|Texas Instruments Incorporated
|XWRL6888 Single-Chip 60GHz mmWave Sensor
[IBIS Ver]   5.0
[File name]   xwrl6888_fccsp329.ibs
[Date]   07/08/2026
[File Rev]   1.0
[Source]   Cadence SpeedXP Suite XtractIM 18.0.4.05011.160686   004
[Notes]   Revision History:
| Rev 1.0: 07/08/2026
| - Initial release of the model.
[Disclaimer]
| This model is designed as an aid for customers of Texas Instruments.
| TI and its licensors and suppliers make no warranties, either expressed
| or implied, with respect to this  model, including the warranties of
| merchantability or fitness for a particular purpose. The model is
| provided solely on an "as is" basis. The entire risk as to its quality
| and performance is with the customer.
| This model is subject to change without notice. Texas Instruments
| Incorporated is not responsible for updating this model.
[Copyright]
(C) Copyright 2021 Texas Instruments Incorporated.All rights reserved.
|  Component AWRL6888DBGAPDRQ1 329-pin FCBGA - APD0329 package
|  Part # AWRL6888DBGAPDRQ1
[Component]   AWRL6888DBGAPDRQ1
[Manufacturer]   Texas Instruments
[Package]   |329 FCCSP - APD0329 package
|  variable   typ   min   max
|   typ   min   max
R_pkg   0.17465   0.069398   0.39969
L_pkg   1.619e-9   6.542e-10   3.167e-9
C_pkg   5.691e-13   3.526e-13   1.287e-12
[Pin]   Signal_name   model_name   R_pin  L_pin  C_pin
A1   VSSA   GND   NA   NA   NA
A2   VSSA   GND   NA   NA   NA
A4   VSSA   GND   NA   NA   NA
A6   VSSA   GND   NA   NA   NA
A8   VSSA   GND   NA   NA   NA
A10   VSSA   GND   NA   NA   NA
A12   VSSA   GND   NA   NA   NA
A14   VSSA   GND   NA   NA   NA
A16   VSSA   GND   NA   NA   NA
A18   VSSA   GND   NA   NA   NA
A19   QSPI_qdin0   IO2   NA   NA   NA
A20   QSPI_qdin1   IO2   NA   NA   NA
A21   VSS   GND   NA   NA   NA
B1   VSSA   GND   NA   NA   NA
B2   VSSA   GND   NA   NA   NA
B3   TX1   NC   NA   NA   NA
B4   VSSA   GND   NA   NA   NA
B5   TX2   NC   NA   NA   NA
B6   VSSA   GND   NA   NA   NA
B7   TX3   NC   NA   NA   NA
B8   VSSA   GND   NA   NA   NA
B9   TX4   NC   NA   NA   NA
B10   VSSA   GND   NA   NA   NA
B11   TX5   NC   NA   NA   NA
B12   VSSA   GND   NA   NA   NA
B13   TX6   NC   NA   NA   NA
B14   VSSA   GND   NA   NA   NA
B15   TX7   NC   NA   NA   NA
B16   VSSA   GND   NA   NA   NA
B17   TX8   NC   NA   NA   NA
B18   VSSA   GND   NA   NA   NA
B19   VSS   GND   NA   NA   NA
B20   VSS   GND   NA   NA   NA
B21   QSPI_din   IO2   NA   NA   NA
C1   VSSA   GND   NA   NA   NA
C2   VSSA   GND   NA   NA   NA
C3   VSSA   GND   NA   NA   NA
C4   VSSA   GND   NA   NA   NA
C5   VSSA   GND   NA   NA   NA
C6   VSSA   GND   NA   NA   NA
C7   VSSA   GND   NA   NA   NA
C8   VSSA   GND   NA   NA   NA
C9   VSSA   GND   NA   NA   NA
C10   VSSA   GND   NA   NA   NA
C11   VSSA   GND   NA   NA   NA
C12   VSSA   GND   NA   NA   NA
C13   VSSA   GND   NA   NA   NA
C14   VSSA   GND   NA   NA   NA
C15   VSSA   GND   NA   NA   NA
C16   VSSA   GND   NA   NA   NA
C17   VSSA   GND   NA   NA   NA
C18   VSSA   GND   NA   NA   NA
C19   SPIA_miso   IO2   NA   NA   NA
C20   QSPI_dout   IO2   NA   NA   NA
C21   QSPI_cs_n   IO2   NA   NA   NA
D1   VSSA   GND   NA   NA   NA
D2   VSSA   GND   NA   NA   NA
D3   VSSA   GND   NA   NA   NA
D4   CLKM   NC   NA   NA   NA
D6   VSSA   GND   NA   NA   NA
D7   VSSA   GND   NA   NA   NA
D8   VSSA   GND   NA   NA   NA
D9   VSSA   GND   NA   NA   NA
D10   VSSA   GND   NA   NA   NA
D11   VSSA   GND   NA   NA   NA
D12   VSSA   GND   NA   NA   NA
D13   VSSA   GND   NA   NA   NA
D14   VSSA   GND   NA   NA   NA
D15   VSSA   GND   NA   NA   NA
D16   VSSA   GND   NA   NA   NA
D17   VSSA   GND   NA   NA   NA
D20   QSPI_clk   IO2   NA   NA   NA
E2   RX8   NC   NA   NA   NA
E3   VSSA   GND   NA   NA   NA
E19   SPIA_mosi   IO2   NA   NA   NA
E20   SPIA_cs0_n   IO2   NA   NA   NA
E21   PMIC_CLKOUT   IO2   NA   NA   NA
F1   VSSA   GND   NA   NA   NA
F2   VSSA   GND   NA   NA   NA
F3   VSSA   GND   NA   NA   NA
F4   CLKP   NC   NA   NA   NA
F6   VOUT_14SYNTH   NC   NA   NA   NA
F8   VDDA_10RF   POWER   NA   NA   NA
F9   VDDA_10RF   POWER   NA   NA   NA
F10   VDDA_10RF   POWER   NA   NA   NA
F11   VDDA_12RF   POWER   NA   NA   NA
F12   VDDA_12RF   POWER   NA   NA   NA
F13   VDDA_12RF   POWER   NA   NA   NA
F14   VSS   GND   NA   NA   NA
F15   VSS   GND   NA   NA   NA
F16   VSS   GND   NA   NA   NA
F19   SPIA_clk   IO2   NA   NA   NA
F20   VSS   GND   NA   NA   NA
F21   VIOIN_18   POWER   NA   NA   NA
G2   RX7   NC   NA   NA   NA
G3   VSSA   GND   NA   NA   NA
G8   VSSA   GND   NA   NA   NA
G9   VSSA   GND   NA   NA   NA
G10   VDD   POWER   NA   NA   NA
G11   VDD   POWER   NA   NA   NA
G12   VDD   POWER   NA   NA   NA
G13   VDD   POWER   NA   NA   NA
G14   VDD   POWER   NA   NA   NA
G15   VDD   POWER   NA   NA   NA
G16   VDD   POWER   NA   NA   NA
G20   VSS   GND   NA   NA   NA
G21   VIOIN   POWER   NA   NA   NA
H1   VSSA   GND   NA   NA   NA
H2   VSSA   GND   NA   NA   NA
H3   VSSA   GND   NA   NA   NA
H4   VSSA   GND   NA   NA   NA
H6   VIOIN_18CLK   POWER   NA   NA   NA
H8   OSC_CLK_OUT   NC   NA   NA   NA
H9   VSSA   GND   NA   NA   NA
H10   VDD   POWER   NA   NA   NA
H11   VDD   POWER   NA   NA   NA
H12   VDD   POWER   NA   NA   NA
H13   VDD   POWER   NA   NA   NA
H14   VDD   POWER   NA   NA   NA
H15   VDD   POWER   NA   NA   NA
H16   VDD   POWER   NA   NA   NA
H19   HOST_CLK_req   IO2   NA   NA   NA
H20   GPIO_2   IO2   NA   NA   NA
J2   RX6   NC   NA   NA   NA
J3   VSSA   GND   NA   NA   NA
J4   VSSA   GND   NA   NA   NA
J8   VSSA   GND   NA   NA   NA
J9   VSSA   GND   NA   NA   NA
J10   VDD   POWER   NA   NA   NA
J11   VDD   POWER   NA   NA   NA
J12   VDD   POWER   NA   NA   NA
J13   VDD   POWER   NA   NA   NA
J14   VDD   POWER   NA   NA   NA
J15   VDD   POWER   NA   NA   NA
J16   VDD   POWER   NA   NA   NA
J19   VSS   GND   NA   NA   NA
J20   LVDS_TXP0   ODF   NA   NA   NA
J21   LVDS_TXM0   ODF   NA   NA   NA
K1   VSSA   GND   NA   NA   NA
K2   VSSA   GND   NA   NA   NA
K3   VSSA   GND   NA   NA   NA
K4   VSSA   GND   NA   NA   NA
K6   VDDA_18VCO   POWER   NA   NA   NA
K8   VOUT_14APLL   NC   NA   NA   NA
K9   VSSA   GND   NA   NA   NA
K10   VDD   POWER   NA   NA   NA
K11   VDD   POWER   NA   NA   NA
K12   VDD   POWER   NA   NA   NA
K13   VDD   POWER   NA   NA   NA
K14   VDD   POWER   NA   NA   NA
K15   VDD   POWER   NA   NA   NA
K16   VDD   POWER   NA   NA   NA
K19   VSS   GND   NA   NA   NA
K20   LVDS_CLKP   ODF   NA   NA   NA
L2   RX5   NC   NA   NA   NA
L3   VSSA   GND   NA   NA   NA
L4   VSSA   GND   NA   NA   NA
L8   VSSA   GND   NA   NA   NA
L9   VSSA   GND   NA   NA   NA
L10   VDD   POWER   NA   NA   NA
L11   VDD   POWER   NA   NA   NA
L12   VDD   POWER   NA   NA   NA
L13   VDD   POWER   NA   NA   NA
L14   VDD   POWER   NA   NA   NA
L15   VDD   POWER   NA   NA   NA
L16   VDD   POWER   NA   NA   NA
L19   VSS   GND   NA   NA   NA
L20   VSS   GND   NA   NA   NA
L21   LVDS_CLKM   ODF   NA   NA   NA
M1   VSSA   GND   NA   NA   NA
M2   VSSA   GND   NA   NA   NA
M3   VSSA   GND   NA   NA   NA
M4   VSSA   GND   NA   NA   NA
M6   VIN_18PM   POWER   NA   NA   NA
M7   VDDA_10RF   POWER   NA   NA   NA
M8   VSSA   GND   NA   NA   NA
M9   VSS   GND   NA   NA   NA
M10   VSS   GND   NA   NA   NA
M11   VSS   GND   NA   NA   NA
M12   VSS   GND   NA   NA   NA
M13   VSS   GND   NA   NA   NA
M14   VSS   GND   NA   NA   NA
M15   VSS   GND   NA   NA   NA
M16   VSS   GND   NA   NA   NA
M19   VIOIN_18LVDS   POWER   NA   NA   NA
M20   VIOIN_18LVDS   POWER   NA   NA   NA
M21   LVDS_FRCLKM   ODF   NA   NA   NA
N2   RX4   NC   NA   NA   NA
N3   VSSA   GND   NA   NA   NA
N4   VSSA   GND   NA   NA   NA
N7   VSSA   GND   NA   NA   NA
N8   VSSA   GND   NA   NA   NA
N9   VSS   GND   NA   NA   NA
N10   VSS   GND   NA   NA   NA
N11   VSS   GND   NA   NA   NA
N12   VSS   GND   NA   NA   NA
N13   VSS   GND   NA   NA   NA
N14   VSS   GND   NA   NA   NA
N15   VSS   GND   NA   NA   NA
N16   VSS   GND   NA   NA   NA
N19   VSS   GND   NA   NA   NA
N20   LVDS_FRCLKP   ODF   NA   NA   NA
P1   VSSA   GND   NA   NA   NA
P2   VSSA   GND   NA   NA   NA
P3   VSSA   GND   NA   NA   NA
P4   VSSA   GND   NA   NA   NA
P6   VBGAP   NC   NA   NA   NA
P7   VSSA   GND   NA   NA   NA
P8   VSSA   GND   NA   NA   NA
P9   VSS   GND   NA   NA   NA
P10   VSS   GND   NA   NA   NA
P11   VSS   GND   NA   NA   NA
P12   VSS   GND   NA   NA   NA
P13   VSS   GND   NA   NA   NA
P14   VSS   GND   NA   NA   NA
P15   VSS   GND   NA   NA   NA
P16   VSS   GND   NA   NA   NA
P19   VSS   GND   NA   NA   NA
P20   LVDS_TXP1   ODF   NA   NA   NA
P21   LVDS_TXM1   ODF   NA   NA   NA
R2   RX3   NC   NA   NA   NA
R3   VSSA   GND   NA   NA   NA
R4   VSSA   GND   NA   NA   NA
R7   VSSA   GND   NA   NA   NA
R8   VSSA   GND   NA   NA   NA
R9   VSS   GND   NA   NA   NA
R10   VSS   GND   NA   NA   NA
R11   VSS   GND   NA   NA   NA
R12   VSS   GND   NA   NA   NA
R13   VSS   GND   NA   NA   NA
R14   VSS   GND   NA   NA   NA
R15   VSS   GND   NA   NA   NA
R16   VSS   GND   NA   NA   NA
R19   VSS   GND   NA   NA   NA
R20   I2C_sda   IO2   NA   NA   NA
T1   VSSA   GND   NA   NA   NA
T2   VSSA   GND   NA   NA   NA
T3   VSSA   GND   NA   NA   NA
T4   VSSA   GND   NA   NA   NA
T7   VSS   GND   NA   NA   NA
T8   VSS   GND   NA   NA   NA
T9   VSS   GND   NA   NA   NA
T10   VSS   GND   NA   NA   NA
T11   VSS   GND   NA   NA   NA
T12   VSS   GND   NA   NA   NA
T13   VSS   GND   NA   NA   NA
T14   VSS   GND   NA   NA   NA
T15   VSS   GND   NA   NA   NA
T16   VSS   GND   NA   NA   NA
T19   VSS   GND   NA   NA   NA
T20   lvds_valid   IO2   NA   NA   NA
T21   I2C_scl   IO2   NA   NA   NA
U2   RX2   NC   NA   NA   NA
U3   VSSA   GND   NA   NA   NA
U4   VSSA   GND   NA   NA   NA
U6   VSS   GND   NA   NA   NA
U7   VSS   GND   NA   NA   NA
U8   VSS   GND   NA   NA   NA
U9   VSS   GND   NA   NA   NA
U10   VSS   GND   NA   NA   NA
U11   VSS   GND   NA   NA   NA
U12   VSS   GND   NA   NA   NA
U13   VSS   GND   NA   NA   NA
U14   VSS   GND   NA   NA   NA
U15   VSS   GND   NA   NA   NA
U16   VSS   GND   NA   NA   NA
U19   VSS   GND   NA   NA   NA
U20   rs232_tx   IO2   NA   NA   NA
U21   sys_reset_out   IO2   NA   NA   NA
V1   VSSA   GND   NA   NA   NA
V2   VSSA   GND   NA   NA   NA
V3   VSSA   GND   NA   NA   NA
V6   VSS   GND   NA   NA   NA
V7   VSS   GND   NA   NA   NA
V8   VSS   GND   NA   NA   NA
V9   VSS   GND   NA   NA   NA
V12   VSS   GND   NA   NA   NA
V13   VSS   GND   NA   NA   NA
V14   VSS   GND   NA   NA   NA
V15   VSS   GND   NA   NA   NA
V16   VSS   GND   NA   NA   NA
V19   VSS   GND   NA   NA   NA
V20   rs232_rx   IO2   NA   NA   NA
W2   RX1   NC   NA   NA   NA
W3   VSSA   GND   NA   NA   NA
W6   VSS   GND   NA   NA   NA
W7   VSS   GND   NA   NA   NA
W8   VSS   GND   NA   NA   NA
W9   VSS   GND   NA   NA   NA
W19   VSS   GND   NA   NA   NA
W20   VSS   GND   NA   NA   NA
W21   VIOIN   POWER   NA   NA   NA
Y1   VSSA   GND   NA   NA   NA
Y2   VSSA   GND   NA   NA   NA
Y3   VSSA   GND   NA   NA   NA
Y4   VDDA_18BB   POWER   NA   NA   NA
Y5   GPADC4   NC   NA   NA   NA
Y6   VPP   POWER   NA   NA   NA
Y7   NRESET   NC   NA   NA   NA
Y8   UARTA_rx   IO1   NA   NA   NA
Y9   VDD   POWER   NA   NA   NA
Y10   VNWA   POWER   NA   NA   NA
Y11   VSS   GND   NA   NA   NA
Y12   VSS   GND   NA   NA   NA
Y13   VDD_SRAM   POWER   NA   NA   NA
Y14   TCK   IO1   NA   NA   NA
Y15   TDO   IO1   NA   NA   NA
Y16   TMS   IO1   NA   NA   NA
Y17   TDI   IO1   NA   NA   NA
Y18   LIN_tx   IO1   NA   NA   NA
Y19   GPIO_5   IO2   NA   NA   NA
Y20   VSS   GND   NA   NA   NA
Y21   VIOIN_18   POWER   NA   NA   NA
AA1   VSSA   GND   NA   NA   NA
AA2   GPADC1   NC   NA   NA   NA
AA3   GPADC2   NC   NA   NA   NA
AA4   VDDA_18BB   POWER   NA   NA   NA
AA6   GPADC3   NC   NA   NA   NA
AA7   UARTA_tx   IO1   NA   NA   NA
AA9   VDD   POWER   NA   NA   NA
AA10   VIOIN_18   POWER   NA   NA   NA
AA12   VIOIN   POWER   NA   NA   NA
AA13   VDD_SRAM   POWER   NA   NA   NA
AA14   CAN_FD_B_tx   IO1   NA   NA   NA
AA16   CAN_FD_B_rx   IO1   NA   NA   NA
AA17   LIN_rx   IO1   NA   NA   NA
AA19   UARTA_rts   IO2   NA   NA   NA
AA20   nERROR_OUT   IO2   NA   NA   NA
AA21   VSS   GND   NA   NA   NA
[Diff Pin]  inv_pin  vdiff  tdelay_typ  tdelay_min  tdelay_max
   P21   P20   0.1   NA   NA   NA
   M21   N20   0.1   NA   NA   NA
   L21   K20   0.1   NA   NA   NA
   J21   J20   0.1   NA   NA   NA
| Model IO1
[Model Selector] IO1
|SC1 IS A SLEW RATE CONTROL PIN
|5% SUPPLY VARIATION MODES WITH 1.8V NOM SUPPLY
IO1_V_PUPDOFF_5P_SC1_1P8  Cell operated at 1.8(nom)
|IO1_V_PUPDOFF_5P_SC1_1P8; BUFFER WITH WEAK PULUP/PULLDOWN OFF AT 5% SUPPLY
|VARIATION WITH SC1=1 MEANING SLOW MODE OF OPERATION
IO1_V_PD_ON_5P_!SC1_1P8  Cell operated at 1.8(nom)
|IO1_V_PD_ON_5P_!SC1_1P8; BUFFER WITH WEAK_PULLDOWN_ON AT 5% SUPPLY
|VARIATION WITH SC1=0 MEANING FAST MODE OF OPERATION
IO1_V_PD_ON_5P_SC1_1P8  Cell operated at 1.8(nom)
|IO1_V_PD_ON_5P_SC1_1P8; BUFFER WITH WEAK_PULLDOWN_ON AT 5% SUPPLY
|VARIATION WITH SC1=1 MEANING SLOW MODE OF OPERATION
IO1_V_PU_ON_5P_!SC1_1P8  Cell operated at 1.8(nom)
|IO1_V_PU_ON_5P_!SC1_1P8; BUFFER WITH WEAK_PULLUP_ON AT 5% SUPPLY
|VARIATION WITH SC1=0 MEANING FAST MODE OF OPERATION
IO1_V_PUPDOFF_5P_!SC1_1P8  Cell operated at 1.8(nom)
|IO1_V_PUPDOFF_5P_!SC1_1P8; BUFFER WITH WEAK PULUP/PULLDOWN OFF AT 5% SUPPLY
|VARIATION WITH SC1=0 MEANING FAST MODE OF OPERATION
IO1_V_PU_ON_5P_SC1_1P8  Cell operated at 1.8(nom)
|IO1_V_PU_ON_5P_SC1_1P8; BUFFER WITH WEAK_PULLUP_ON AT 5% SUPPLY
|VARIATION WITH SC1=1 MEANING SLOW MODE OF OPERATION
|5% SUPPLY VARIATION MODES WITH 3.3V NOM SUPPLY
IO1_V_PUPDOFF_5P_SC1_3P3  Cell operated at 3.3(nom)
|IO1_V_PUPDOFF_5P_SC1_3P3; BUFFER WITH WEAK PULUP/PULLDOWN OFF AT 5% SUPPLY
|VARIATION WITH SC1=1 MEANING SLOW MODE OF OPERATION
IO1_V_PD_ON_5P_!SC1_3P3  Cell operated at 3.3(nom)
|IO1_V_PD_ON_5P_!SC1_3P3; BUFFER WITH WEAK_PULLDOWN_ON AT 5% SUPPLY
|VARIATION WITH SC1=0 MEANING FAST MODE OF OPERATION
IO1_V_PD_ON_5P_SC1_3P3  Cell operated at 3.3(nom)
|IO1_V_PD_ON_5P_SC1_3P3; BUFFER WITH WEAK_PULLDOWN_ON AT 5% SUPPLY
|VARIATION WITH SC1=1 MEANING SLOW MODE OF OPERATION
IO1_V_PU_ON_5P_!SC1_3P3  Cell operated at 3.3(nom)
|IO1_V_PU_ON_5P_!SC1_3P3; BUFFER WITH WEAK_PULLUP_ON AT 5% SUPPLY
|VARIATION WITH SC1=0 MEANING FAST MODE OF OPERATION
IO1_V_PUPDOFF_5P_!SC1_3P3  Cell operated at 3.3(nom)
|IO1_V_PUPDOFF_5P_!SC1_3P3; BUFFER WITH WEAK PULUP/PULLDOWN OFF AT 5% SUPPLY
|VARIATION WITH SC1=0 MEANING FAST MODE OF OPERATION
IO1_V_PU_ON_5P_SC1_3P3  Cell operated at 3.3(nom)
|IO1_V_PU_ON_5P_SC1_3P3; BUFFER WITH WEAK_PULLUP_ON AT 5% SUPPLY
|VARIATION WITH SC1=1 MEANING SLOW MODE OF OPERATION
| 10% SUPPLY VARIATION MODES WITH 1.8V NOM SUPPLY
IO1_V_PUPDOFF_10P_SC1_1P8  Cell operated at 1.8(nom)
|IO1_V_PUPDOFF_10P_SC1_1P8; BUFFER WITH WEAK PULUP/PULLDOWN OFF AT 10% SUPPLY
|VARIATION WITH SC1=1 MEANING SLOW MODE OF OPERATION
IO1_V_PD_ON_10P_!SC1_1P8  Cell operated at 1.8(nom)
|IO1_V_PD_ON_10P_!SC1_1P8; BUFFER WITH WEAK_PULLDOWN_ON AT 10% SUPPLY
|VARIATION WITH SC1=0 MEANING FAST MODE OF OPERATION
IO1_V_PD_ON_10P_SC1_1P8  Cell operated at 1.8(nom)
|IO1_V_PD_ON_10P_SC1_1P8; BUFFER WITH WEAK_PULLDOWN_ON AT 10% SUPPLY
|VARIATION WITH SC1=1 MEANING SLOW MODE OF OPERATION
IO1_V_PU_ON_10P_!SC1_1P8  Cell operated at 1.8(nom)
|IO1_V_PU_ON_10P_!SC1_1P8; BUFFER WITH WEAK_PULLUP_ON AT 10% SUPPLY
|VARIATION WITH SC1=0 MEANING FAST MODE OF OPERATION
IO1_V_PUPDOFF_10P_!SC1_1P8  Cell operated at 1.8(nom)
|IO1_V_PUPDOFF_10P_!SC1_1P8; BUFFER WITH WEAK PULUP/PULLDOWN OFF AT 10% SUPPLY
|VARIATION WITH SC1=0 MEANING FAST MODE OF OPERATION
IO1_V_PU_ON_10P_SC1_1P8  Cell operated at 1.8(nom)
|IO1_V_PU_ON_10P_SC1_1P8; BUFFER WITH WEAK_PULLUP_ON AT 10% SUPPLY
|VARIATION WITH SC1=1 MEANING SLOW MODE OF OPERATION
| 10% SUPPLY VARIATION MODES WITH 3.3V NOM SUPPLY
IO1_V_PUPDOFF_10P_SC1_3P3  Cell operated at 3.3(nom)
|IO1_V_PUPDOFF_10P_SC1_3P3; BUFFER WITH WEAK PULUP/PULLDOWN OFF AT 10% SUPPLY
|VARIATION WITH SC1=1 MEANING SLOW MODE OF OPERATION
IO1_V_PD_ON_10P_!SC1_3P3  Cell operated at 3.3(nom)
|IO1_V_PD_ON_10P_!SC1_3P3; BUFFER WITH WEAK_PULLDOWN_ON 10% SUPPLY
|VARIATION WITH SC1=0 MEANING FAST MODE OF OPERATION
IO1_V_PD_ON_10P_SC1_3P3  Cell operated at 3.3(nom)
|IO1_V_PD_ON_10P_SC1_3P3; BUFFER WITH WEAK_PULLDOWN_ON AT 10% SUPPLY
|VARIATION WITH SC1=1 MEANING SLOW MODE OF OPERATION
IO1_V_PU_ON_10P_!SC1_3P3  Cell operated at 3.3(nom)
|IO1_V_PU_ON_10P_!SC1_3P3; BUFFER WITH WEAK_PULLUP_ON AT 10% SUPPLY
|VARIATION WITH SC1=0 MEANING FAST MODE OF OPERATION
IO1_V_PUPDOFF_10P_!SC1_3P3  Cell operated at 3.3(nom)
|IO1_V_PUPDOFF_10P_!SC1_3P3; BUFFER WITH WEAK PULUP/PULLDOWN OFF AT 10% SUPPLY
|VARIATION WITH SC1=0 MEANING FAST MODE OF OPERATION
IO1_V_PU_ON_10P_SC1_3P3  Cell operated at 3.3(nom)
|IO1_V_PU_ON_10P_SC1_3P3; BUFFER WITH WEAK_PULLUP_ON AT 10% SUPPLY
|VARIATION WITH SC1=1 MEANING SLOW MODE OF OPERATION
| Model IO2
[Model Selector] IO2
|SC1 IS A SLEW RATE CONTROL PIN
|5% SUPPLY VARIATION MODES WITH 1.8V NOM SUPPLY
IO2_H_PUPDOFF_5P_SC1_1P8  Cell operated at 1.8(nom)
|IO2_H_PUPDOFF_5P_SC1_1P8; BUFFER WITH WEAK PULUP/PULLDOWN OFF AT 5% SUPPLY
|VARIATION WITH SC1=1 MEANING SLOW MODE OF OPERATION
IO2_H_PD_ON_5P_!SC1_1P8  Cell operated at 1.8(nom)
|IO2_H_PD_ON_5P_!SC1_1P8; BUFFER WITH WEAK_PULLDOWN_ON AT 5% SUPPLY
|VARIATION WITH SC1=0 MEANING FAST MODE OF OPERATION
IO2_H_PD_ON_5P_SC1_1P8  Cell operated at 1.8(nom)
|IO2_H_PD_ON_5P_SC1_1P8; BUFFER WITH WEAK_PULLDOWN_ON AT 5% SUPPLY
|VARIATION WITH SC1=1 MEANING SLOW MODE OF OPERATION
IO2_H_PU_ON_5P_!SC1_1P8  Cell operated at 1.8(nom)
|IO2_H_PU_ON_5P_!SC1_1P8; BUFFER WITH WEAK_PULLUP_ON AT 5% SUPPLY
|VARIATION WITH SC1=0 MEANING FAST MODE OF OPERATION
IO2_H_PUPDOFF_5P_!SC1_1P8  Cell operated at 1.8(nom)
|IO2_H_PUPDOFF_5P_!SC1_1P8; BUFFER WITH WEAK PULUP/PULLDOWN OFF AT 5% SUPPLY
|VARIATION WITH SC1=0 MEANING FAST MODE OF OPERATION
IO2_H_PU_ON_5P_SC1_1P8  Cell operated at 1.8(nom)
|IO2_H_PU_ON_5P_SC1_1P8; BUFFER WITH WEAK_PULLUP_ON AT 5% SUPPLY
|VARIATION WITH SC1=1 MEANING SLOW MODE OF OPERATION
|5% SUPPLY VARIATION MODES WITH 3.3V NOM SUPPLY
IO2_H_PUPDOFF_5P_SC1_3P3  Cell operated at 3.3(nom)
|IO2_H_PUPDOFF_5P_SC1_3P3; BUFFER WITH WEAK PULUP/PULLDOWN OFF AT 5% SUPPLY
|VARIATION WITH SC1=1 MEANING SLOW MODE OF OPERATION
IO2_H_PD_ON_5P_!SC1_3P3  Cell operated at 3.3(nom)
|IO2_H_PD_ON_5P_!SC1_3P3; BUFFER WITH WEAK_PULLDOWN_ON AT 5% SUPPLY
|VARIATION WITH SC1=0 MEANING FAST MODE OF OPERATION
IO2_H_PD_ON_5P_SC1_3P3  Cell operated at 3.3(nom)
|IO2_H_PD_ON_5P_SC1_3P3; BUFFER WITH WEAK_PULLDOWN_ON AT 5% SUPPLY
|VARIATION WITH SC1=1 MEANING SLOW MODE OF OPERATION
IO2_H_PU_ON_5P_!SC1_3P3  Cell operated at 3.3(nom)
|IO2_H_PU_ON_5P_!SC1_3P3; BUFFER WITH WEAK_PULLUP_ON AT 5% SUPPLY
|VARIATION WITH SC1=0 MEANING FAST MODE OF OPERATION
IO2_H_PUPDOFF_5P_!SC1_3P3  Cell operated at 3.3(nom)
|IO2_H_PUPDOFF_5P_!SC1_3P3; BUFFER WITH WEAK PULUP/PULLDOWN OFF AT 5% SUPPLY
|VARIATION WITH SC1=0 MEANING FAST MODE OF OPERATION
IO2_H_PU_ON_5P_SC1_3P3  Cell operated at 3.3(nom)
|IO2_H_PU_ON_5P_SC1_3P3; BUFFER WITH WEAK_PULLUP_ON AT 5% SUPPLY
|VARIATION WITH SC1=1 MEANING SLOW MODE OF OPERATION
| 10% SUPPLY VARIATION MODES WITH 1.8V NOM SUPPLY
IO2_H_PUPDOFF_10P_SC1_1P8  Cell operated at 1.8(nom)
|IO2_H_PUPDOFF_10P_SC1_1P8; BUFFER WITH WEAK PULUP/PULLDOWN OFF AT 10% SUPPLY
|VARIATION WITH SC1=1 MEANING SLOW MODE OF OPERATION
IO2_H_PD_ON_10P_!SC1_1P8  Cell operated at 1.8(nom)
|IO2_H_PD_ON_10P_!SC1_1P8; BUFFER WITH WEAK_PULLDOWN_ON AT 10% SUPPLY
|VARIATION WITH SC1=0 MEANING FAST MODE OF OPERATION
IO2_H_PD_ON_10P_SC1_1P8  Cell operated at 1.8(nom)
|IO2_H_PD_ON_10P_SC1_1P8; BUFFER WITH WEAK_PULLDOWN_ON AT 10% SUPPLY
|VARIATION WITH SC1=1 MEANING SLOW MODE OF OPERATION
IO2_H_PU_ON_10P_!SC1_1P8  Cell operated at 1.8(nom)
|IO2_H_PU_ON_10P_!SC1_1P8; BUFFER WITH WEAK_PULLUP_ON AT 10% SUPPLY
|VARIATION WITH SC1=0 MEANING FAST MODE OF OPERATION
IO2_H_PUPDOFF_10P_!SC1_1P8  Cell operated at 1.8(nom)
|IO2_H_PUPDOFF_10P_!SC1_1P8; BUFFER WITH WEAK PULUP/PULLDOWN OFF AT 10% SUPPLY
|VARIATION WITH SC1=0 MEANING FAST MODE OF OPERATION
IO2_H_PU_ON_10P_SC1_1P8  Cell operated at 1.8(nom)
|IO2_H_PU_ON_10P_SC1_1P8; BUFFER WITH WEAK_PULLUP_ON AT 10% SUPPLY
|VARIATION WITH SC1=1 MEANING SLOW MODE OF OPERATION
| 10% SUPPLY VARIATION MODES WITH 3.3V NOM SUPPLY
IO2_H_PUPDOFF_10P_SC1_3P3  Cell operated at 3.3(nom)
|IO2_H_PUPDOFF_10P_SC1_3P3; BUFFER WITH WEAK PULUP/PULLDOWN OFF AT 10% SUPPLY
|VARIATION WITH SC1=1 MEANING SLOW MODE OF OPERATION
IO2_H_PD_ON_10P_!SC1_3P3  Cell operated at 3.3(nom)
|IO2_H_PD_ON_10P_!SC1_3P3; BUFFER WITH WEAK_PULLDOWN_ON 10% SUPPLY
|VARIATION WITH SC1=0 MEANING FAST MODE OF OPERATION
IO2_H_PD_ON_10P_SC1_3P3  Cell operated at 3.3(nom)
|IO2_H_PD_ON_10P_SC1_3P3; BUFFER WITH WEAK_PULLDOWN_ON AT 10% SUPPLY
|VARIATION WITH SC1=1 MEANING SLOW MODE OF OPERATION
IO2_H_PU_ON_10P_!SC1_3P3  Cell operated at 3.3(nom)
|IO2_H_PU_ON_10P_!SC1_3P3; BUFFER WITH WEAK_PULLUP_ON AT 10% SUPPLY
|VARIATION WITH SC1=0 MEANING FAST MODE OF OPERATION
IO2_H_PUPDOFF_10P_!SC1_3P3  Cell operated at 3.3(nom)
|IO2_H_PUPDOFF_10P_!SC1_3P3; BUFFER WITH WEAK PULUP/PULLDOWN OFF AT 10% SUPPLY
|VARIATION WITH SC1=0 MEANING FAST MODE OF OPERATION
IO2_H_PU_ON_10P_SC1_3P3  Cell operated at 3.3(nom)
|IO2_H_PU_ON_10P_SC1_3P3; BUFFER WITH WEAK_PULLUP_ON AT 10% SUPPLY
|VARIATION WITH SC1=1 MEANING SLOW MODE OF OPERATION
| Model ODF
[Model Selector] ODF
ODF_MODE_10P_1P8  Cell operated at 1.8(nom)
|ODF_MODE_10P_1P8; LVDS DRIVER MODE WITH 10PER VDDS
ODF_MODE_5P_1P8  Cell operated at 1.8(nom)
[Define Package Model]   AWRL6888DBGAPDRQ1
[Manufacturer]   TI
[OEM]   TI
[Description]   FCBGA
|[Number of Sections]   1
[Number of Pins]   64
[Pin Numbers]
|[Pin Name]  Net Number   Net Name   Net's All Pins
D4   | 1   CLKM   D4
F4   | 2   CLKP   F4
H8   | 3   OSC_CLK_OUT   H8
P6   | 4   VBGAP   P6
AA9   | 5   VDD   AA9
   |G10
   |G11
   |G12
   |G13
   |G14
   |G15
   |G16
   |H10
   |H11
   |H12
   |H13
   |H14
   |H15
   |H16
   |J10
   |J11
   |J12
   |J13
   |J14
   |J15
   |J16
   |K10
   |K11
   |K12
   |K13
   |K14
   |K15
   |K16
   |L10
   |L11
   |L12
   |L13
   |L14
   |L15
   |L16
   |Y9
F8   | 6   VDDA_10RF   F8
   |F9
   |F10
   |M7
F11   | 7   VDDA_12RF   F11
   |F12
   |F13
AA4   | 8   VDDA_18BB   AA4
   |Y4
K6   | 9   VDDA_18VCO   K6
AA13   | 10   VDD_SRAM   AA13
   |Y13
M6   | 11   VIN_18PM   M6
AA12   | 12   VIOIN   AA12
   |G21
   |W21
AA10   | 13   VIOIN_18   AA10
   |F21
   |Y21
H6   | 14   VIOIN_18CLK   H6
M19   | 15   VIOIN_18LVDS   M19
   |M20
Y10   | 16   VNWA   Y10
K8   | 17   VOUT_14APLL   K8
F6   | 18   VOUT_14SYNTH   F6
Y6   | 19   VPP   Y6
AA16   | 20   CAN_FD_B_RX   AA16
AA14   | 21   CAN_FD_B_TX   AA14
AA2   | 22   GPADC1   AA2
AA3   | 23   GPADC2   AA3
AA6   | 24   GPADC3   AA6
Y5   | 25   GPADC4   Y5
H20   | 26   GPIO_2   H20
Y19   | 27   GPIO_5   Y19
H19   | 28   HOST_CLK_REQ   H19
T21   | 29   I2C_SCL   T21
R20   | 30   I2C_SDA   R20
AA17   | 31   LIN_RX   AA17
Y18   | 32   LIN_TX   Y18
L21   | 33   LVDS_CLKM   L21
K20   | 34   LVDS_CLKP   K20
M21   | 35   LVDS_FRCLKM   M21
N20   | 36   LVDS_FRCLKP   N20
J21   | 37   LVDS_TXM0   J21
P21   | 38   LVDS_TXM1   P21
J20   | 39   LVDS_TXP0   J20
P20   | 40   LVDS_TXP1   P20
T20   | 41   LVDS_VALID   T20
AA20   | 42   NERROR_OUT   AA20
Y7   | 43   NRESET   Y7
E21   | 44   PMIC_CLKOUT   E21
D20   | 45   QSPI_CLK   D20
C21   | 46   QSPI_CS_N   C21
B21   | 47   QSPI_DIN   B21
C20   | 48   QSPI_DOUT   C20
A19   | 49   QSPI_QDIN0   A19
A20   | 50   QSPI_QDIN1   A20
V20   | 51   RS232_RX   V20
U20   | 52   RS232_TX   U20
F19   | 53   SPIA_CLK   F19
E20   | 54   SPIA_CS0_N   E20
C19   | 55   SPIA_MISO   C19
E19   | 56   SPIA_MOSI   E19
U21   | 57   SYS_RESET_OUT   U21
Y14   | 58   TCK   Y14
Y17   | 59   TDI   Y17
Y15   | 60   TDO   Y15
Y16   | 61   TMS   Y16
AA19   | 62   UARTA_RTS   AA19
Y8   | 63   UARTA_RX   Y8
AA7   | 64   UARTA_TX   AA7
[Model Data]
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[End Model Data]
[End Package Model]
| Models and submodels in the file (50): IO1_V_PUPDOFF_5P_SC1_1P8 (I/O), IO1_V_PD_ON_5P_!SC1_1P8 (I/O), IO1_V_PD_ON_5P_SC1_1P8 (I/O), IO1_V_PU_ON_5P_!SC1_1P8 (I/O), IO1_V_PUPDOFF_5P_!SC1_1P8 (I/O), IO1_V_PU_ON_5P_SC1_1P8 (I/O), IO1_V_PUPDOFF_5P_SC1_3P3 (I/O), IO1_V_PD_ON_5P_!SC1_3P3 (I/O), IO1_V_PD_ON_5P_SC1_3P3 (I/O), IO1_V_PU_ON_5P_!SC1_3P3 (I/O), IO1_V_PUPDOFF_5P_!SC1_3P3 (I/O), IO1_V_PU_ON_5P_SC1_3P3 (I/O), IO1_V_PUPDOFF_10P_SC1_1P8 (I/O), IO1_V_PD_ON_10P_!SC1_1P8 (I/O), IO1_V_PD_ON_10P_SC1_1P8 (I/O), IO1_V_PU_ON_10P_!SC1_1P8 (I/O), IO1_V_PUPDOFF_10P_!SC1_1P8 (I/O), IO1_V_PU_ON_10P_SC1_1P8 (I/O), IO1_V_PUPDOFF_10P_SC1_3P3 (I/O), IO1_V_PD_ON_10P_!SC1_3P3 (I/O), IO1_V_PD_ON_10P_SC1_3P3 (I/O), IO1_V_PU_ON_10P_!SC1_3P3 (I/O), IO1_V_PUPDOFF_10P_!SC1_3P3 (I/O), IO1_V_PU_ON_10P_SC1_3P3 (I/O), IO2_H_PUPDOFF_5P_SC1_1P8 (I/O), IO2_H_PD_ON_5P_!SC1_1P8 (I/O), IO2_H_PD_ON_5P_SC1_1P8 (I/O), IO2_H_PU_ON_5P_!SC1_1P8 (I/O), IO2_H_PUPDOFF_5P_!SC1_1P8 (I/O), IO2_H_PU_ON_5P_SC1_1P8 (I/O), IO2_H_PUPDOFF_5P_SC1_3P3 (I/O), IO2_H_PD_ON_5P_!SC1_3P3 (I/O), IO2_H_PD_ON_5P_SC1_3P3 (I/O), IO2_H_PU_ON_5P_!SC1_3P3 (I/O), IO2_H_PUPDOFF_5P_!SC1_3P3 (I/O), IO2_H_PU_ON_5P_SC1_3P3 (I/O), IO2_H_PUPDOFF_10P_SC1_1P8 (I/O), IO2_H_PD_ON_10P_!SC1_1P8 (I/O), IO2_H_PD_ON_10P_SC1_1P8 (I/O), IO2_H_PU_ON_10P_!SC1_1P8 (I/O), IO2_H_PUPDOFF_10P_!SC1_1P8 (I/O), IO2_H_PU_ON_10P_SC1_1P8 (I/O), IO2_H_PUPDOFF_10P_SC1_3P3 (I/O), IO2_H_PD_ON_10P_!SC1_3P3 (I/O), IO2_H_PD_ON_10P_SC1_3P3 (I/O), IO2_H_PU_ON_10P_!SC1_3P3 (I/O), IO2_H_PUPDOFF_10P_!SC1_3P3 (I/O), IO2_H_PU_ON_10P_SC1_3P3 (I/O), ODF_MODE_10P_1P8 (3-state), ODF_MODE_5P_1P8 (3-state)
